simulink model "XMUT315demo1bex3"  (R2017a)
settings: Solver=VariableStepAuto  StartTime=0.0  StopTime=10.0  RelTol=1e-3
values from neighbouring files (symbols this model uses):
  Dm = 0.2    [XMUT315democomplexmodel.m]
  Jm = 0.02    [XMUT315democomplexmodel.m]
  Kb = 0.1    [XMUT315democomplexmodel.m]
  Kt = 0.1    [XMUT315democomplexmodel.m]
  La = 0.5    [XMUT315democomplexmodel.m]
  Ra = 2    [XMUT315democomplexmodel.m]

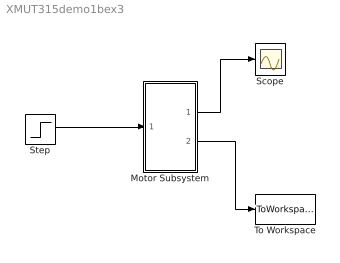
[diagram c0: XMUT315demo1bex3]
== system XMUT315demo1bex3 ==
  Motor Subsystem : Subsystem
  Scope : Scope
  Step : Step  Time=2  SampleTime=0
  To Workspace : ToWorkspace  VariableName=simout  SaveFormat=Timeseries  SampleTime=-1
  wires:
  Step/1 -> Motor Subsystem/1(In1)
  Motor Subsystem/1(Out1) -> Scope/1
  Motor Subsystem/2(Out2) -> To Workspace/1

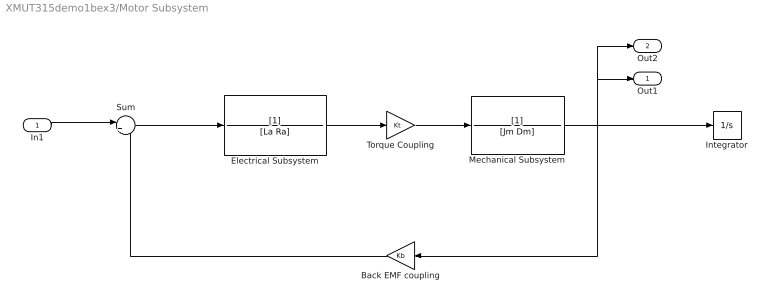
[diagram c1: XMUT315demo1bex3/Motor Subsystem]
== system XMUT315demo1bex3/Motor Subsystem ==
  In1 : Inport
  Back EMF coupling : Gain  Gain=Kb
  Electrical Subsystem : TransferFcn  Denominator=[La Ra]
  Integrator : Integrator
  Mechanical Subsystem : TransferFcn  Denominator=[Jm Dm]
  Sum : Sum  Inputs=|+-
  Torque Coupling : Gain  Gain=Kt
  Out1 : Outport
  Out2 : Outport  Port=2
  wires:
  Mechanical Subsystem/1 -> Out2/1, Out1/1, Integrator/1, Back EMF coupling/1
  Electrical Subsystem/1 -> Torque Coupling/1
  Back EMF coupling/1 -> Sum/2
  Torque Coupling/1 -> Mechanical Subsystem/1
  Sum/1 -> Electrical Subsystem/1
  In1/1 -> Sum/1
